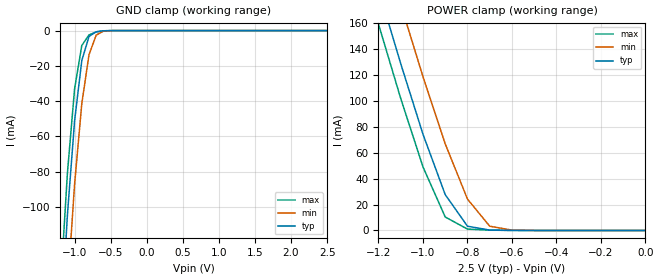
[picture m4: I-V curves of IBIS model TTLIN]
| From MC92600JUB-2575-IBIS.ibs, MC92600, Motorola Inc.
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|   Model TTLIN
[Model]   TTLIN
Model_type   Input
Vinl =   0.8000V
Vinh =   2.0000V
C_comp   4.3400pF   NA   NA
[Temperature Range]   40.0000   0.1050k   0.000
[Pullup Reference]   2.5000V   2.3000V   2.7000V
[Pulldown Reference]   0.000V   0.000V   0.000V
[POWER Clamp Reference]   2.5000V   2.3000V   2.7000V
[GND Clamp Reference]   0.000V   0.000V   0.000V
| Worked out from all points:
|   GND clamp passes 1 mA (typ) near -0.71 V on its own axis
|   POWER clamp passes 1 mA (typ) near -0.72 V on its own axis
[GND_clamp]
| voltage   I(typ)   I(min)   I(max)
-2.5V     -1.395A    -1.435A    -1.373A
-1.2V     -175.2mA   -221.4mA   -148.8mA
-1.1V     -104.9mA   -148mA     -81.11mA
-1V       -51.16mA   -87.12mA   -33.03mA
-900mV    -17.02mA   -41.39mA   -8.438mA
-800mV    -3.316mA   -13.66mA   -2.451mA
-700mV    -667.4uA   -2.555mA   -759.1uA
-600mV    -130.7uA   -310.5uA   -127.8uA
2.5V      1.267nA    182.7nA    86.7nA
[POWER_clamp]
| voltage   I(typ)   I(min)   I(max)
-2.5V     988.6mA    1.03A      964.9mA
-1.2V     186mA      232mA      159mA
-1.1V     128.5mA    174.2mA    101.7mA
-1V       74.15mA    118.5mA    48.99mA
-900mV    27.61mA    66.69mA    10.37mA
-800mV    3.292mA    24.21mA    1.065mA
-700mV    291.1uA    3.285mA    251.6uA
-600mV    49.84uA    254.7uA    43.18uA
0V        1.267nA    69.31nA    94.89nA
